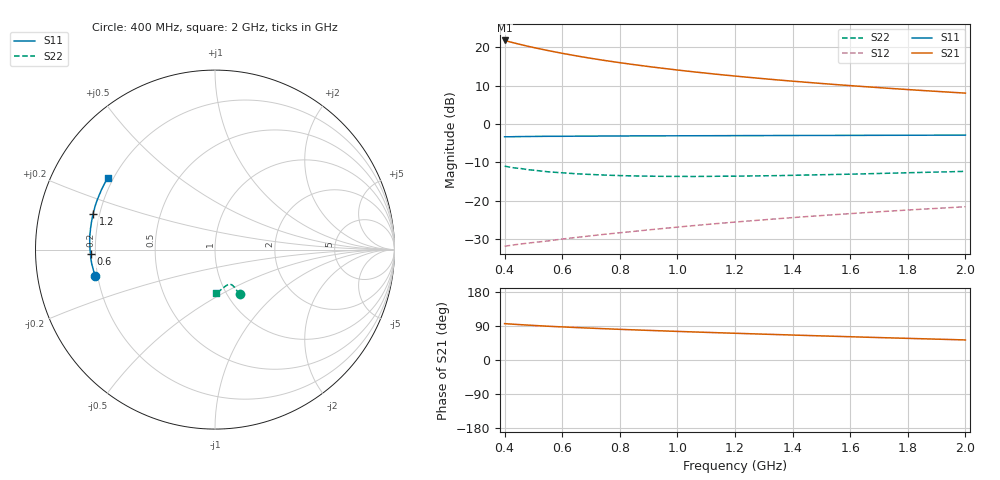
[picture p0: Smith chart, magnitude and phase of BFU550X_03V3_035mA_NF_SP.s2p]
! Filename:  P:\Prog\Test\Noise\ATS_data\Testdata_Net\bfu550X de embed 3currents\BFU550X_APG2013_44_C05_03p3V_035mA_NF_CM01_D.sf
! Date/Time: Mon 29/Jul/2013 14:56:12
! BFU550X_APG2013_44_C05_03p3V_1to35mA_NF_CM01_Bias8_R.sf
! Noise Parameter Data File
! BFU550X_APG2013_44_C05_03p3V_1to35mA_NF_CM01
! Date/time: Fri Jul 19 17:23:25 2013
! VAR V_out= 3.300000
! VAR I_out= 34.995000
! VAR V_in= 0.844400
! VAR I_in= 0.414500
! Device data file deembeded for feedlines and parallel
! Original file: \bfu550X de embed 3currents\BFU550X_APG2013_44_C05_03p3V_035mA_NF_CM01_R.sf
! Feed-files: PR005V01_100713_Feed1.s2p, PR005V01_100713_Feed2.s2p
! Parallel-file: PR005V01_100713_Par.s2p
# MHz S MA R 50
!  Freq-MHz  S11-mag  S11-arg  S21-mag  S21-arg  S12-mag  S12-arg  S22-mag  S22-arg
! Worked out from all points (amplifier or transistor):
!   37 points, 400 MHz to 2 GHz, reference 50 ohm
!   highest |S21| = 21.8 dB at 400 MHz (marker M1)
!   |S21| within 3 dB of that: start of sweep to 576 MHz
!   unconditionally stable (mu >= 1): 821.6 MHz to end of sweep
!   at 500 MHz: K = 0.84, MSG = 25.4 dB, |S12| = -30.9 dB
!   at 1.1 GHz: K = 1.06, MAG = 18.3 dB, |S12| = -26.2 dB
!   at 2 GHz: K = 1.09, MAG = 13.0 dB, |S12| = -21.5 dB
!   lowest NFmin = 1.31 dB at 750 MHz
!   S11 on the Smith chart (normalised r, x): 400 MHz: 0.19, -0.10; 600 MHz: 0.18, -0.02; 1.2 GHz: 0.17, +0.14; 2 GHz: 0.18, +0.29
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400  0.6836 -167.6  12.32 96.0  0.02564 49.2  0.283 -60.9
420  0.684 -168.9  11.76 94.9  0.02623 49.8  0.2743 -61.4
440  0.6868 -170.1  11.26 94.0  0.02689 50.4  0.267 -61.3
480  0.6894 -172.3  10.37 92.2  0.02806 51.3  0.2549 -62.1
500  0.6911 -173.4  9.976 91.2  0.02862 51.7  0.251 -62.1
550  0.6938 -175.9  9.111 89.1  0.02998 53.4  0.2391 -62.5
600  0.6938 -178.0  8.377 87.3  0.03175 54.6  0.2319 -63.0
650  0.6966 -179.9  7.746 85.6  0.03336 55.6  0.2253 -63.5
700  0.6972 178.2  7.206 84.0  0.03499 56.6  0.2203 -64.1
750  0.6992 176.5  6.734 82.4  0.03671 57.5  0.2165 -64.8
800  0.7011 174.9  6.324 80.9  0.03834 58.3  0.2133 -65.6
850  0.7019 173.3  5.958 79.5  0.04 59.1  0.2111 -66.3
900  0.7022 171.8  5.629 78.1  0.04181 59.9  0.2096 -67.0
950  0.7034 170.4  5.339 76.8  0.04359 60.5  0.2086 -67.8
1050  0.7048 167.7  4.833 74.2  0.04727 61.6  0.2078 -69.5
1100  0.7057 166.4  4.615 73.0  0.04914 62.0  0.2082 -70.4
1200  0.7076 163.9  4.233 70.5  0.05284 62.6  0.2097 -72.2
1350  0.7102 160.2  3.763 67.0  0.05851 63.4  0.213 -75.2
1500  0.7123 156.8  3.388 63.6  0.06425 63.8  0.2189 -78.1
1600  0.7133 154.6  3.176 61.4  0.06809 63.9  0.2226 -80.1
1750  0.7153 151.3  2.902 58.2  0.07396 63.9  0.2297 -83.2
2000  0.719 146.2  2.535 52.9  0.08369 63.8  0.2422 -88.1
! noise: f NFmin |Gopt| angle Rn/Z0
400  1.39  0.4055  -172.2  0.0775
460  1.339  0.434  -170.5  0.0701
600  1.349  0.4571  -167.8  0.0663
800  1.377  0.5065  -164.3  0.0581
1000  1.409  0.5321  -160.7  0.0585
1200  1.448  0.5469  -157.8  0.0649
1400  1.472  0.581  -153.2  0.0722
1600  1.514  0.6245  -149.4  0.0784
1800  1.539  0.6045  -146.3  0.098
2000  1.585  0.6324  -142.5  0.1196
